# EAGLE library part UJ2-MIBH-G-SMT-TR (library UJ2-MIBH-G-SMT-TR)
USB Connectors Source: Datasheet
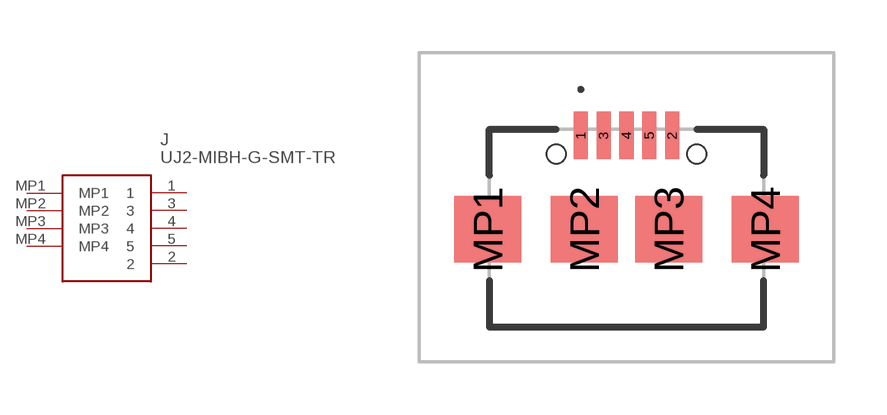
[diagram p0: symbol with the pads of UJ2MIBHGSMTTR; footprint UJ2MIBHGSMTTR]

Designator prefix J

## UJ2-MIBH-G-SMT-TR (Arrow_Part_Number: UJ2-MIBH-G-SMT-TR; Arrow_Price-Stock: https://www.arrow.com/en/products/uj2-mibh-g-smt-tr/cui-devices?region=nac; Description: USB Connectors; Height: 3.15mm; Manufacturer_Name: CUI Inc.; Manufacturer_Part_Number: UJ2-MIBH-G-SMT-TR; Mouser_Part_Number: 490-UJ2-MIBH-G-SMTTR; Mouser_Price-Stock: https://www.mouser.co.uk/ProductDetail/CUI-Devices/UJ2-MIBH-G-SMT-TR?qs=IS%252B4QmGtzzpvS1XQusp0iA%3D%3D)  [UJ2MIBHGSMTTR]
1  1
2  2
3  3
4  4
5  5
MP1  MP1
MP2  MP2
MP3  MP3
MP4  MP4

## Footprint UJ2MIBHGSMTTR (pad centres in mm)
UJ2-MIBH-G-SMT-TR-2
smd 0.4 x 1.35: 1 -1.3,2.64; 2 1.3,2.64; 3 -0.65,2.64; 4 0,2.64; 5 0.65,2.64
smd 1.9 x 1.9: MP1 -3.95,-0.035; MP2 -1.2,-0.035; MP3 1.2,-0.035; MP4 3.95,-0.035
hole 0.55 at -2,2.115
hole 0.55 at 2,2.115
